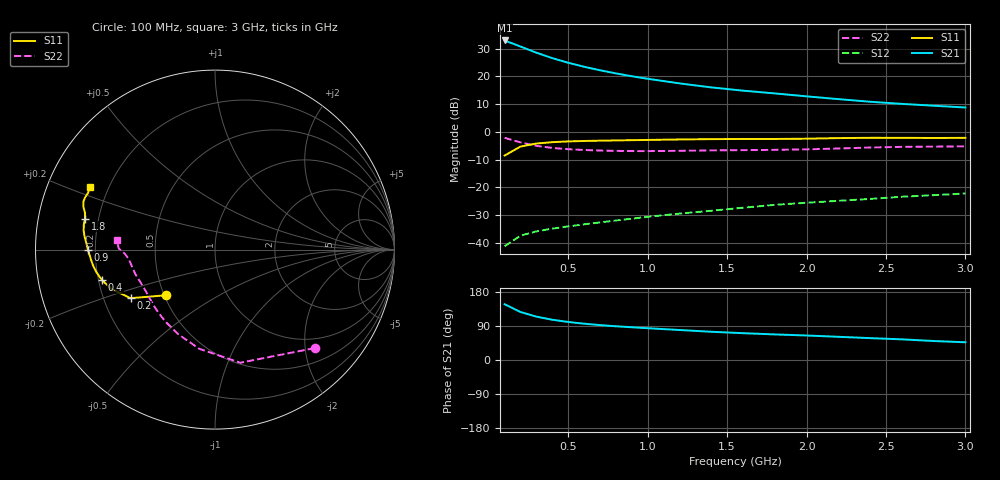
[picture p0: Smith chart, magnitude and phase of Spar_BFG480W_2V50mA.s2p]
! Filename: 250BFG480.001
! Title: BFG480W
! Bias: Vce=2V; Ic=50mA
! Company: NXP Semiconductors NL
! User: Quality&Reliability T&D
! Measure time: 10 Nov 1999 / 11:54:01
#  MHz  S  MA  R 50
! Freq  S11  S21  S12  S22  :
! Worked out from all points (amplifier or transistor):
!   20 points, 100 MHz to 3 GHz, reference 50 ohm
!   highest |S21| = 32.9 dB at 100 MHz (marker M1)
!   |S21| within 3 dB of that: start of sweep to 236.6 MHz
!   unconditionally stable (mu >= 1): 915.5 MHz to end of sweep
!   at 400 MHz: K = 0.66, MSG = 30.7 dB, |S12| = -34.9 dB
!   at 1.2 GHz: K = 1.06, MAG = 21.9 dB, |S12| = -29.5 dB
!   at 3 GHz: K = 1.11, MAG = 13.5 dB, |S12| = -22.2 dB
!   S11 on the Smith chart (normalised r, x): 100 MHz: 0.51, -0.30; 200 MHz: 0.32, -0.24; 400 MHz: 0.21, -0.13; 900 MHz: 0.17, +0.00; 1.8 GHz: 0.15, +0.12; 3 GHz: 0.13, +0.23
100  0.374 -137.1  44.32 147.2  0.008712 67.3  0.7809 -44.6
200  0.5431 -150.1  34.46 126.7  0.01351 55.2  0.6458 -77.4
300  0.6156 -159.0  26.67 114.4  0.01609 51.5  0.5595 -99.0
400  0.6516 -164.8  21.28 106.2  0.01804 51.3  0.5131 -113.9
500  0.6723 -169.1  17.59 100.3  0.01979 52.6  0.487 -124.6
600  0.6848 -172.5  14.88 95.8  0.02155 54.2  0.4712 -132.5
700  0.6932 -175.3  12.88 92.2  0.02335 56.2  0.4607 -138.6
800  0.7002 -177.8  11.31 89.0  0.02525 58.2  0.4538 -143.6
900  0.7082 180.0  10.05 86.4  0.02723 60.3  0.4504 -147.9
1000  0.7146 178.0  9.049 83.9  0.02944 61.7  0.4497 -151.7
1200  0.7291 174.5  7.474 79.2  0.03363 64.1  0.4552 -157.8
1400  0.7392 171.9  6.328 74.5  0.03789 65.8  0.4634 -162.4
1600  0.7439 169.3  5.526 70.8  0.04294 67.3  0.468 -165.9
1800  0.7442 166.5  4.927 67.5  0.04839 68.4  0.4739 -169.6
2000  0.7527 164.2  4.36 64.7  0.0528 69.5  0.4837 -173.7
2200  0.7716 161.9  3.888 61.2  0.05717 69.9  0.501 -177.1
2400  0.7805 160.0  3.485 57.7  0.06185 69.7  0.5217 -179.3
2600  0.7802 158.2  3.191 54.5  0.06777 69.4  0.5361 179.2
2800  0.7749 155.9  2.957 50.1  0.07231 68.2  0.5418 177.3
3000  0.7793 153.2  2.747 46.8  0.07748 67.7  0.5483 174.4
